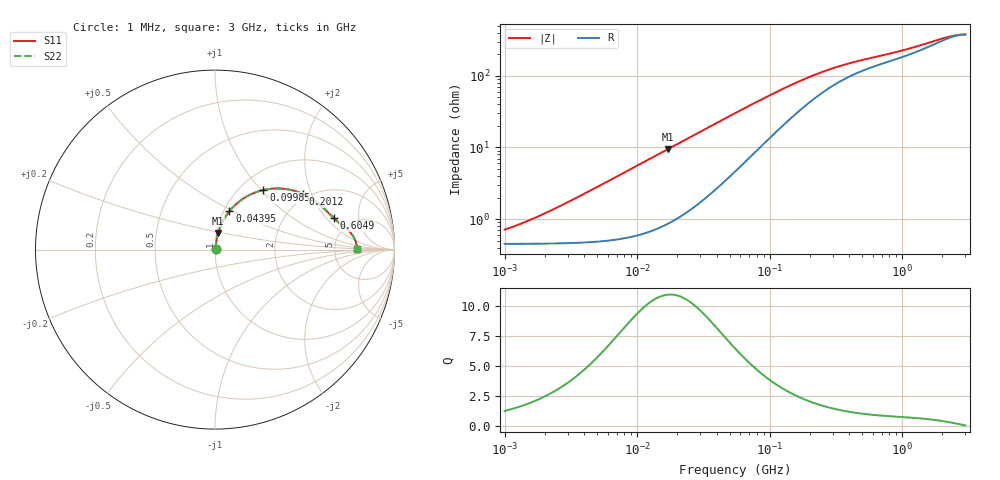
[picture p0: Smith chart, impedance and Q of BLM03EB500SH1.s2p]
! BLM03EB500SH1
# Hz S RI R 50
!Freq.(Hz) S11(Real) S11(Imag) S21(Real) S21(Imag) S12(Real) S12(Imag) S22(Real) S22(Imag)
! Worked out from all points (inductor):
!   401 points, 1 MHz to 3 GHz, reference 50 ohm
!   read as one part in series: L = 88.2 nH near 2.511 MHz
!   highest Q = 11 at 17.15 MHz (marker M1), where L = 88.1 nH
!   S11 on the Smith chart (normalised r, x): 1 MHz: 1.01, +0.01; 43.95 MHz: 1.06, +0.48; 99.85 MHz: 1.27, +1.03; 201.2 MHz: 1.86, +1.74; 604.9 MHz: 3.68, +2.42; 3 GHz: 8.54, +0.14
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1000000  0.00452 0.00549  0.9955 -0.00549  0.9955 -0.00549  0.00452 0.00549
1271492  0.00455 0.00699  0.9954 -0.00699  0.9954 -0.00699  0.00455 0.00699
1751453  0.00462 0.00962  0.9954 -0.00962  0.9954 -0.00962  0.00462 0.00962
3823119  0.00513 0.021  0.9949 -0.021  0.9949 -0.021  0.00513 0.021
8017732  0.00732 0.0439  0.9927 -0.0439  0.9927 -0.0439  0.00732 0.0439
1.461624e7  0.0138 0.0792  0.9862 -0.0792  0.9862 -0.0792  0.0138 0.0792
1.71545e7  0.0173 0.0925  0.9827 -0.0925  0.9827 -0.0925  0.0173 0.0925
2.886629e7  0.0395 0.1503  0.9605 -0.1503  0.9605 -0.1503  0.0395 0.1503
4.394807e7  0.0804 0.2142  0.9196 -0.2142  0.9196 -0.2142  0.0804 0.2142
5.477226e7  0.1153 0.2513  0.8847 -0.2513  0.8847 -0.2513  0.1153 0.2513
7.248696e7  0.1769 0.296  0.8231 -0.296  0.8231 -0.296  0.1769 0.296
9.984923e7  0.2696 0.332  0.7304 -0.332  0.7304 -0.332  0.2696 0.332
1.403209e8  0.3812 0.339  0.6188 -0.339  0.6188 -0.339  0.3812 0.339
2.011837e8  0.4891 0.3103  0.5109 -0.3103  0.5109 -0.3103  0.4891 0.3103
2.094008e8  0.4996 0.3055  0.5004 -0.3055  0.5004 -0.3055  0.4996 0.3055
2.609752e8  0.5501 0.2761  0.4499 -0.2761  0.4499 -0.2761  0.5501 0.2761
3.318279e8  0.5929 0.2425  0.4071 -0.2425  0.4071 -0.2425  0.5929 0.2425
6.049187e8  0.6624 0.1744  0.3376 -0.1744  0.3376 -0.1744  0.6624 0.1744
8.005644e8  0.6882 0.152  0.3118 -0.152  0.3118 -0.152  0.6882 0.152
1.45942e9  0.7467 0.1039  0.2533 -0.1039  0.2533 -0.1039  0.7467 0.1039
2.266846e9  0.7823 0.0488  0.2177 -0.0488  0.2177 -0.0488  0.7823 0.0488
3e9  0.7903 0.00317  0.2097 -0.00317  0.2097 -0.00317  0.7903 0.00317
